(* Logix 5000 Rung export; software revision 20.03 *)

TYPE GSCEthernetType :   // Allows read/write Ethernet settings between the module and processor
STRUCT
   Read : BOOL;   // Enable Ethernet configuration transfer from module to processor
   Write : BOOL;   // Enable Ethernet configuration transfer from processor to module
   Config : GSCEthernet;
END_STRUCT
END_TYPE

TYPE GSCDateTime :   // Stores the date and time value
STRUCT
   Year : DINT;
   Month : DINT;
   Day : DINT;
   Hour : DINT;
   Minute : DINT;
   Seconds : DINT;
END_STRUCT
END_TYPE

TYPE GSCEthernet :   // Stores the MVI56-MCM IP settings
STRUCT
   IP : INT[4];
   Netmask : INT[4];
   Gateway : INT[4];
END_STRUCT
END_TYPE

TYPE GSCClockType :   // Allows read/write of clock value between the module and processor
STRUCT
   Read : BOOL;   // Reads current time from the module
   Write : BOOL;   // Writes current time from the module
   Config : GSCDateTime;   // Date and time configuration read or written between the module and processor
END_STRUCT
END_TYPE

ADD_ON_INSTRUCTION AOI69EGSC_Optional   (* revision 1.0 *)
// MVI69E-GSC Optional Add-On Ethernet/Clock.
// Revision note:
// Release AOI
VAR_IN_OUT
   MVI69EGSCEthernet : GSCEthernetType; {required}   // MVI56E-MCM Rev2 Ethernet Settings
   MVI69EGSCClock : GSCClockType; {required}   // MVI56E-MCM Rev2 Clock Settings
   ReadEthernetMSG : MESSAGE; {required}   // Read Ethernet Settings Message
   WriteEthernetMSG : MESSAGE; {required}   // Write Ethernet Settings Message
   ReadClockMSG : MESSAGE; {required}   // Read Clock Settings Message
   WriteClockMSG : MESSAGE; {required}   // Write Clock Settings Message
END_VAR

ROUTINE Logic   (* ladder *)
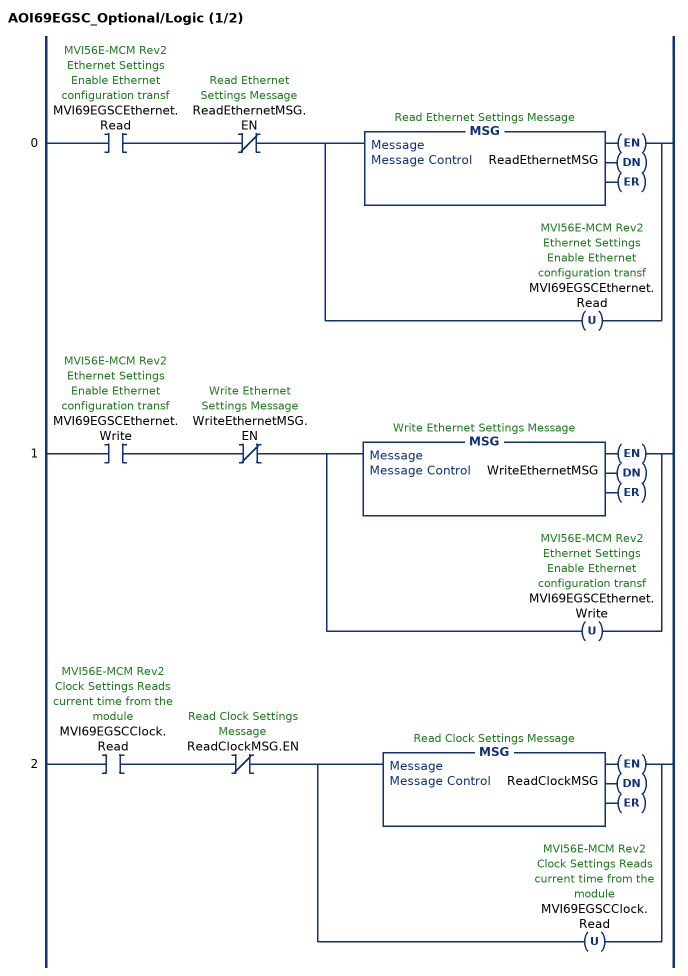
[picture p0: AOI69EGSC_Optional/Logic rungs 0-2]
   0: XIC(MVI69EGSCEthernet.Read)XIO(ReadEthernetMSG.EN)[MSG(ReadEthernetMSG) ,OTU(MVI69EGSCEthernet.Read) ];
   1: XIC(MVI69EGSCEthernet.Write)XIO(WriteEthernetMSG.EN)[MSG(WriteEthernetMSG) ,OTU(MVI69EGSCEthernet.Write) ];
   2: XIC(MVI69EGSCClock.Read)XIO(ReadClockMSG.EN)[MSG(ReadClockMSG) ,OTU(MVI69EGSCClock.Read) ];
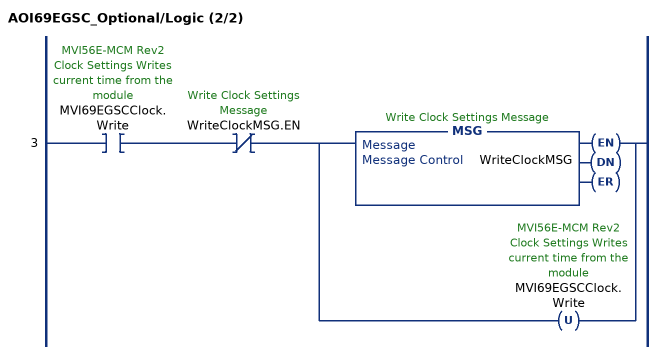
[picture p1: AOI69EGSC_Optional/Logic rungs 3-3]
   3: XIC(MVI69EGSCClock.Write)XIO(WriteClockMSG.EN)[MSG(WriteClockMSG) ,OTU(MVI69EGSCClock.Write) ];
END_ROUTINE
END_ADD_ON_INSTRUCTION

VAR_GLOBAL   (* controller tags *)
   WriteClockMSG : MESSAGE;
        MessageParameters(MessageType := CIP Generic, RequestedLength := 24, ConnectedFlag := 2, ConnectionPath := GSC, ServiceCode := 16#0010, ObjectType := 16#00c7, TargetObject := 8, AttributeNumber := 16#0020, LocalElement := MVI69EGSCClock.Config)
   ReadEthernetMSG : MESSAGE;
        MessageParameters(MessageType := CIP Generic, ConnectedFlag := 2, ConnectionPath := GSC, ServiceCode := 16#000e, ObjectType := 16#00c7, TargetObject := 8, AttributeNumber := 16#0010, DestinationTag := MVI69EGSCEthernet.Config)
   WriteEthernetMSG : MESSAGE;
        MessageParameters(MessageType := CIP Generic, RequestedLength := 24, ConnectedFlag := 2, ConnectionPath := GSC, ServiceCode := 16#0010, ObjectType := 16#00c7, TargetObject := 8, AttributeNumber := 16#0010, LocalElement := MVI69EGSCEthernet.Config)
   ReadClockMSG : MESSAGE;
        MessageParameters(MessageType := CIP Generic, ConnectedFlag := 2, ConnectionPath := GSC, ServiceCode := 16#000e, ObjectType := 16#00c7, TargetObject := 8, AttributeNumber := 16#0020, DestinationTag := MVI69EGSCClock.Config)
   MVI69EGSCClock : GSCClockType := (Config.Year := 2021, Config.Month := 7, Config.Day := 20, Config.Hour := 11, Config.Minute := 26, Config.Seconds := 29);
   AOI69EGSC_Optional : AOI69EGSC_Optional;
   MVI69EGSCEthernet : GSCEthernetType := (Config.IP[0] := 192, Config.IP[1] := 168, Config.IP[3] := 255, Config.Netmask[0] := 255, Config.Netmask[1] := 255, Config.Netmask[2] := 255, Config.Gateway[0] := 192, Config.Gateway[1] := 168, Config.Gateway[3] := 1);
END_VAR

PROGRAM MainProgram

ROUTINE MainRoutine   (* ladder *)
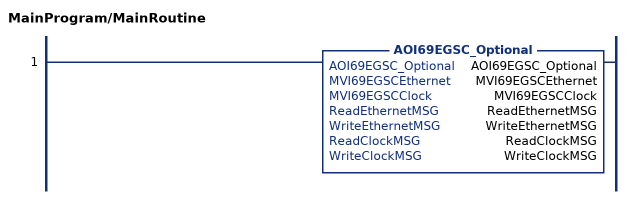
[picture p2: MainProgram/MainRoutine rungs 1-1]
   1: AOI69EGSC_Optional(AOI69EGSC_Optional,MVI69EGSCEthernet,MVI69EGSCClock,ReadEthernetMSG,WriteEthernetMSG,ReadClockMSG,WriteClockMSG);
END_ROUTINE
END_PROGRAM
